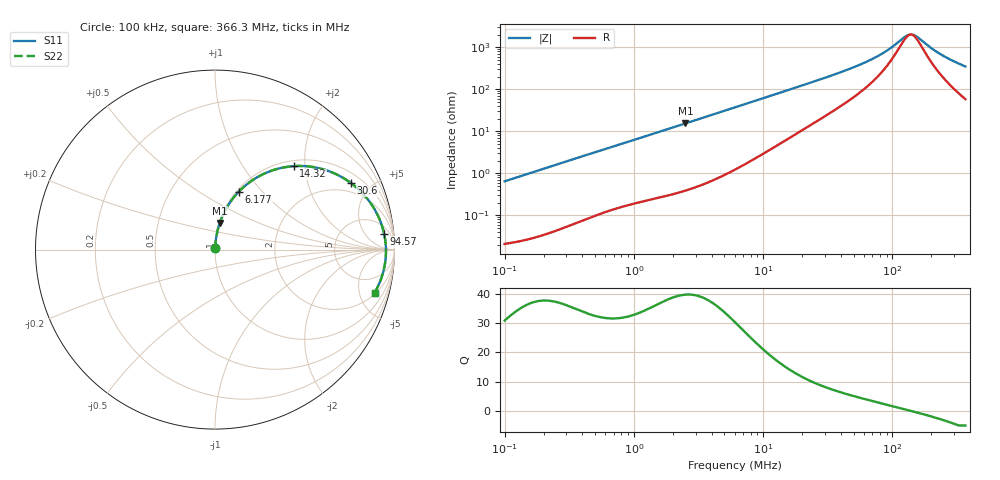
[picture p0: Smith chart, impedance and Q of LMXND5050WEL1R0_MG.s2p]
! LMXND5050WEL1R0_MG  S-PARAMETER MODEL  ( General Type )
! Model Generated by TAIYO YUDEN Corporation (http://www.ty-top.com)
! Version 1.0
! TAIYO YUDEN Control No. 191023NI43SB-FBB
! Copyright(c) 2019 TAIYO YUDEN CO.,LTD. All Rights Reserved.
! Product Description (link to TY-COMPAS)
! https://ds.yuden.co.jp/TYCOMPAS/or/detail?pn=LMXND5050WEL1R0NMG&u=M
! Products Name : Inductors
! Characteristics :
!  Inductance : 1.0 uH , SRF(min) : 85 MHz , DC Resistance(max) : 0.0192 Ohm
!  Rated Current : Saturation :5800 mA , Temp Rise : 4400 mA
!  Case Size : 4.9 x 4.9 / 0.193 x 0.193 [mm/inch] , Thickness : 2.5 / 0.098 [mm/inch]
!  (Conditions: Temperature = 25 degC , DC Bias Current/Voltage = 0A / 0V)
! External Node Assignments :
!  1  o---GGG---o  2
! GND o---------o GND
! Frequency Range : 0.1MHz  -  366.261039MHz  [ 402 STEP ]
# MHz S RI R 50
! Freq[MHz].  S11 Real  S11 Imag  S21 Real  S21 Imag  S12 Real  S12 Imag  S22 Real  S22 Imag
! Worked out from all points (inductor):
!   401 points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, 100 kHz to 366.3 MHz, reference 50 ohm
!   read as one part in series: L = 1.02 uH near 104.2 kHz
!   highest Q = 39.8 at 2.505 MHz (marker M1), where L = 974 nH
!   self-resonance near 138.5 MHz
!   S11 on the Smith chart (normalised r, x): 100 kHz: 1.00, +0.01; 6.177 MHz: 1.03, +0.75; 14.32 MHz: 1.11, +1.75; 30.6 MHz: 1.47, +3.79; 94.57 MHz: 10, +16; 366.3 MHz: 2.16, -6.85
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0.1  0.000248 0.0064  0.9998 -0.0064  0.9998 -0.0064  0.000248 0.0064
0.395307  0.00136 0.025  0.9986 -0.025  0.9986 -0.025  0.00136 0.025
1.562679  0.0117 0.0947  0.9883 -0.0947  0.9883 -0.0947  0.0117 0.0947
2.504885  0.0265 0.1486  0.9735 -0.1486  0.9735 -0.1486  0.0265 0.1486
4.098409  0.0645 0.2325  0.9355 -0.2325  0.9355 -0.2325  0.0645 0.2325
6.177387  0.1326 0.3229  0.8674 -0.3229  0.8674 -0.3229  0.1326 0.3229
9.121891  0.2463 0.4093  0.7537 -0.4093  0.7537 -0.4093  0.2463 0.4093
14.32496  0.4381 0.465  0.5619 -0.465  0.5619 -0.465  0.4381 0.465
23.92381  0.6693 0.4229  0.3307 -0.4229  0.3307 -0.4229  0.6693 0.4229
30.60159  0.7582 0.3704  0.2418 -0.3704  0.2418 -0.3704  0.7582 0.3704
41.62806  0.841 0.2925  0.159 -0.2925  0.159 -0.2925  0.841 0.2925
58.99936  0.9016 0.2019  0.0984 -0.2019  0.0984 -0.2019  0.9016 0.2019
77.03188  0.9294 0.1357  0.0706 -0.1357  0.0706 -0.1357  0.9294 0.1357
94.57258  0.9427 0.0871  0.0573 -0.0871  0.0573 -0.0871  0.9427 0.0871
126.037  0.9518 0.0214  0.0482 -0.0214  0.0482 -0.0214  0.9518 0.0214
134.0375  0.9524 0.00748  0.0476 -0.00748  0.0476 -0.00748  0.9524 0.00748
142.5459  0.9527 -0.00645  0.0473 0.00645  0.0473 0.00645  0.9527 -0.00645
154.7365  0.9523 -0.0251  0.0477 0.0251  0.0477 0.0251  0.9523 -0.0251
197.9276  0.9464 -0.0822  0.0536 0.0822  0.0536 0.0822  0.9464 -0.0822
238.0629  0.9366 -0.127  0.0634 0.127  0.0634 0.127  0.9366 -0.127
298.3293  0.9168 -0.185  0.0832 0.185  0.0832 0.185  0.9168 -0.185
366.261  0.889 -0.2407  0.111 0.2407  0.111 0.2407  0.889 -0.2407
